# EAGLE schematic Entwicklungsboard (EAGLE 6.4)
Projekt einer Entwicklungsplatine. Designed vom Denys Maiier. Fakultät der Naturwissenschaften und Technik der HAWK Göttingen.

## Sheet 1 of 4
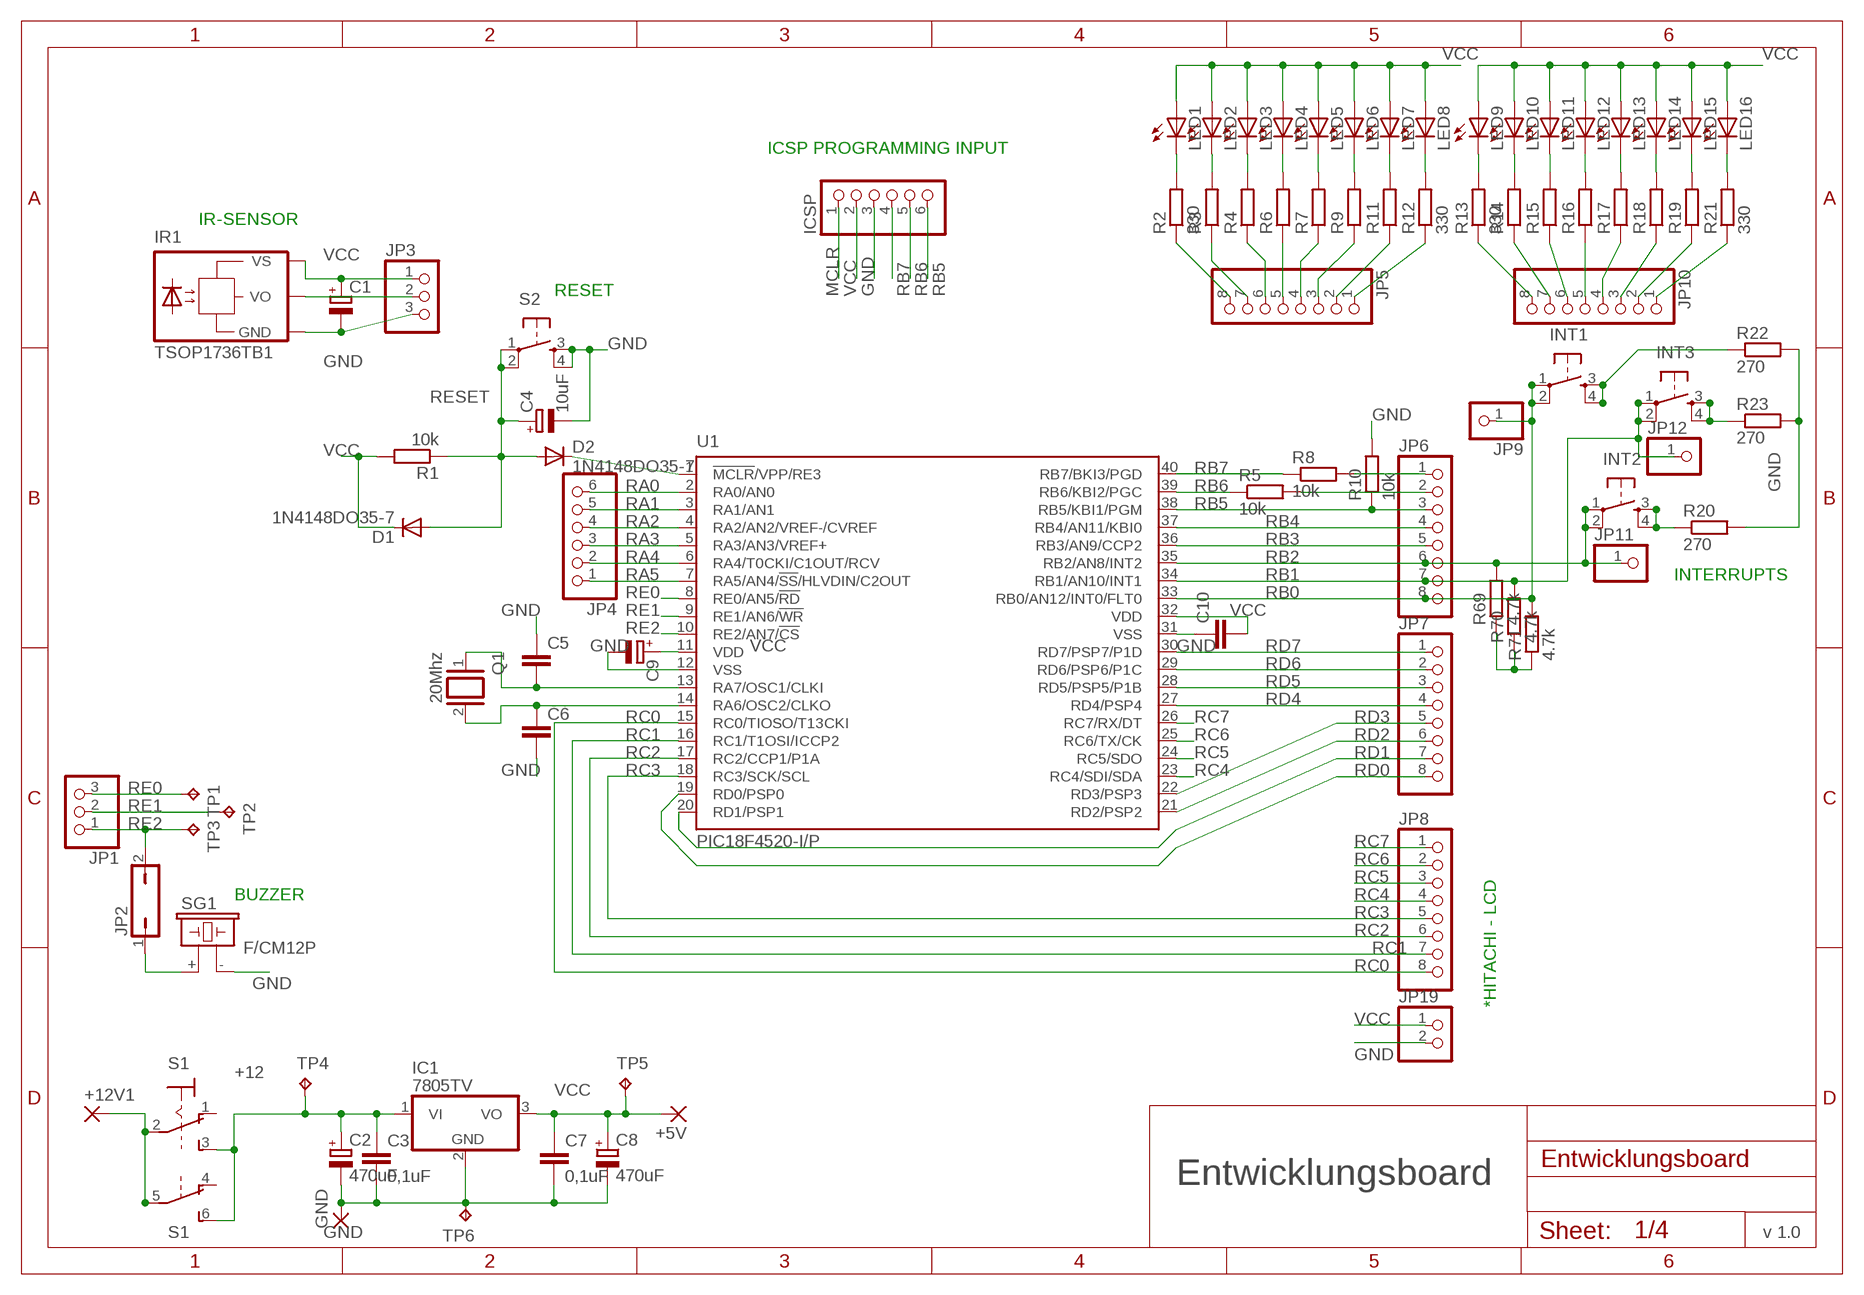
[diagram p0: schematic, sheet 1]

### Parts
+5V  2,15/1,0  [2,15/1,0]
+12V1  2,15/1,0  [2,15/1,0]
C1  CPOL-EUE2.5-5  [E2,5-5]
C2  470uF  CPOL-EUE7.5-16  [E7,5-16]
C3  0,1uF  C-EU075-042X103  [C075-042X103]
C4  10uF  CPOL-EUE2.5-6  [E2,5-6]
C5  C-EUC0805  [C0805]
C6  C-EUC0805  [C0805]
C7  0,1uF  C-EU075-042X103  [C075-042X103]
C8  470uF  CPOL-EUE7.5-16  [E7,5-16]
C9  CPOL-EUE3.5-8  [E3,5-8]
C10  C-EU050-025X075  [C050-025X075]
D1  1N4148DO35-7  [DO35-7]
D2  1N4148DO35-7  [DO35-7]
GND  2,15/1,0  [2,15/1,0]
IC1  7805TV  [TO220V]
ICSP  PINHD-1X6  [1X06]
INT1  10-XXB3FRAFI  [RAFI]
INT2  10-XXB3FRAFI  [RAFI]
INT3  10-XXB3FRAFI  [RAFI]
IR1  TSOP1736TB1  [TSOP17_TB1]
JP1  PINHD-1X3/90  [1X03/90]
JP2  JP1Q  [JP1]
JP3  PINHD-1X3  [1X03]
JP4  PINHD-1X6  [1X06]
JP5  PINHD-1X8  [1X08]
JP6  PINHD-1X8  [1X08]
JP7  PINHD-1X8  [1X08]
JP8  PINHD-1X8  [1X08]
JP9  PINHD-1X1  [1X01]
JP10  PINHD-1X8  [1X08]
JP11  PINHD-1X1  [1X01]
JP12  PINHD-1X1  [1X01]
JP19  PINHD-1X2  [1X02]
LED1  LED5MM  [LED5MM]
LED2  LED5MM  [LED5MM]
LED3  LED5MM  [LED5MM]
LED4  LED5MM  [LED5MM]
LED5  LED5MM  [LED5MM]
LED6  LED5MM  [LED5MM]
LED7  LED5MM  [LED5MM]
LED8  LED5MM  [LED5MM]
LED9  LED5MM  [LED5MM]
LED10  LED5MM  [LED5MM]
LED11  LED5MM  [LED5MM]
LED12  LED5MM  [LED5MM]
LED13  LED5MM  [LED5MM]
LED14  LED5MM  [LED5MM]
LED15  LED5MM  [LED5MM]
LED16  LED5MM  [LED5MM]
Q1  20Mhz  XTAL/S  [QS]
R1  10k  R-EU_M0805  [M0805]
R2  330  R-EU_M0805  [M0805]
R3  R-EU_M0805  [M0805]
R4  R-EU_M0805  [M0805]
R5  10k  R-EU_M0805  [M0805]
R6  R-EU_M0805  [M0805]
R7  R-EU_M0805  [M0805]
R8  10k  R-EU_M0805  [M0805]
R9  R-EU_M0805  [M0805]
R10  10k  R-EU_M0805  [M0805]
R11  R-EU_M0805  [M0805]
R12  330  R-EU_M0805  [M0805]
R13  330  R-EU_M0805  [M0805]
R14  R-EU_M0805  [M0805]
R15  R-EU_M0805  [M0805]
R16  R-EU_M0805  [M0805]
R17  R-EU_M0805  [M0805]
R18  R-EU_M0805  [M0805]
R19  R-EU_M0805  [M0805]
R20  270  R-EU_M0805  [M0805]
R21  330  R-EU_M0805  [M0805]
R22  270  R-EU_M0805  [M0805]
R23  270  R-EU_M0805  [M0805]
R69  4.7k  R-EU_M0805  [M0805]
R70  4.7k  R-EU_M0805  [M0805]
R71  4.7k  R-EU_M0805  [M0805]
S1  320-938  [320-938]
S2  10-XXB3FRAFI  [RAFI]
SG1  F/CM12P  [F/CM12P]
TP1  TPB2,54  [B2,54]
TP2  TPB2,54  [B2,54]
TP3  TPB2,54  [B2,54]
TP4  TPB2,54  [B2,54]
TP5  TPB2,54  [B2,54]
TP6  TPB2,54  [B2,54]
U1  PIC18F4520-I/P  [DIL40]

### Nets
+12: C2.+ C3.1 IC1.1(VI) S1.3(1:S) S1.6(B:S) TP4.TP
GND [GND]: C1.- C2.- C3.2 C4.- C5.1 C6.2 C7.2 C8.- C9.- C10.1 GND.1(P) IC1.2(GND) ICSP.3 IR1.GND JP3.3 JP19.2 R10.2 R20.2 R22.2 R23.2 S2.3(S) S2.4(S1) SG1.- TP6.TP U1.12(VSS) U1.31(VSS)
MCLR: D2.C ICSP.1 U1.1(!MCLR!/VPP/RE3)
N$1: C5.2 Q1.1 U1.13(RA7/OSC1/CLKI)
N$2: JP5.8 R2.1
N$3: C6.1 Q1.2 U1.14(RA6/OSC2/CLKO)
N$4: JP5.7 R3.1
N$5: JP10.8 R13.1
N$6: JP10.7 R14.1
N$7: JP10.6 R15.1
N$8: JP10.5 R16.1
N$9: JP10.4 R17.1
N$10: JP10.3 R18.1
N$11: JP10.2 R19.1
N$12: JP10.1 R21.1
N$13: LED9.K(C) R13.2
N$14: LED11.K(C) R15.2
N$15: LED12.K(C) R16.2
N$16: LED13.K(C) R17.2
N$17: LED16.K(C) R21.2
N$18: LED14.K(C) R18.2
N$19: LED10.K(C) R14.2
N$20: LED15.K(C) R19.2
N$21: JP5.6 R4.1
N$22: JP5.5 R6.1
N$23: JP5.4 R7.1
N$24: JP5.3 R9.1
N$25: JP5.2 R11.1
N$26: JP5.1 R12.1
N$27: LED1.K(C) R2.2
N$28: LED3.K(C) R4.2
N$29: LED4.K(C) R6.2
N$30: LED5.K(C) R7.2
N$31: LED8.K(C) R12.2
N$32: LED2.K(C) R3.2
N$33: LED6.K(C) R9.2
N$34: LED7.K(C) R11.2
N$48: INT1.3(S) INT1.4(S1) R22.1
N$57: JP6.1 R8.2
N$66: JP6.2 R5.2
N$118: INT2.3(S) INT2.4(S1) R20.1
N$122: JP2.1 SG1.+
N$137: IR1.VO JP3.2
N$160: INT3.3(S) INT3.4(S1) R23.1
N$163: +12V1.1(P) S1.2(1:P) S1.5(B:P)
RA0: JP4.6 U1.2(RA0/AN0)
RA1: JP4.5 U1.3(RA1/AN1)
RA2: JP4.4 U1.4(RA2/AN2/VREF-/CVREF)
RA3: JP4.3 U1.5(RA3/AN3/VREF+)
RA4: JP4.2 U1.6(RA4/T0CKI/C1OUT/RCV)
RA5: JP4.1 U1.7(RA5/AN4/!SS!/HLVDIN/C2OUT)
RB0: INT1.1(P) INT1.2(P1) JP6.8 JP9.1 R71.2 U1.33(RB0/AN12/INT0/FLT0)
RB1: INT3.1(P) INT3.2(P1) JP6.7 JP12.1 R70.2 U1.34(RB1/AN10/INT1)
RB2: INT2.1(P) INT2.2(P1) JP6.6 JP11.1 R69.2 U1.35(RB2/AN8/INT2)
RB3: JP6.5 U1.36(RB3/AN9/CCP2)
RB4: JP6.4 U1.37(RB4/AN11/KBI0)
RB5: ICSP.6 JP6.3 R10.1 U1.38(RB5/KBI1/PGM)
RB6: ICSP.5 R5.1 U1.39(RB6/KBI2/PGC)
RB7: ICSP.4 R8.1 U1.40(RB7/BKI3/PGD)
RC0: JP8.8 U1.15(RC0/TIOSO/T13CKI)
RC1: JP8.7 U1.16(RC1/T1OSI/ICCP2)
RC2: JP8.6 U1.17(RC2/CCP1/P1A)
RC3: JP8.5 U1.18(RC3/SCK/SCL)
RC4: JP8.4 U1.23(RC4/SDI/SDA)
RC5: JP8.3 U1.24(RC5/SDO)
RC6: JP8.2 U1.25(RC6/TX/CK)
RC7: JP8.1 U1.26(RC7/RX/DT)
RD0: JP7.8 U1.19(RD0/PSP0)
RD1: JP7.7 U1.20(RD1/PSP1)
RD2: JP7.6 U1.21(RD2/PSP2)
RD3: JP7.5 U1.22(RD3/PSP3)
RD4: JP7.4 U1.27(RD4/PSP4)
RD5: JP7.3 U1.28(RD5/PSP5/P1B)
RD6: JP7.2 U1.29(RD6/PSP6/P1C)
RD7: JP7.1 U1.30(RD7/PSP7/P1D)
RE0: JP1.3 TP1.TP U1.8(RE0/AN5/!RD)
RE1: JP1.2 TP2.TP U1.9(RE1/AN6/!WR)
RE2: JP1.1 JP2.2 TP3.TP U1.10(RE2/AN7/!CS)
RESET: C4.+ D1.A D2.A R1.1 S2.1(P) S2.2(P1)
VCC [VCC]: +5V.1(P) C1.+ C7.1 C8.+ C9.+ C10.2 D1.C IC1.3(VO) ICSP.2 IR1.VS JP3.1 JP19.1 LED1.A LED2.A LED3.A LED4.A LED5.A LED6.A LED7.A LED8.A LED9.A LED10.A LED11.A LED12.A LED13.A LED14.A LED15.A LED16.A R1.2 R69.1 R70.1 R71.1 TP5.TP U1.11(VDD) U1.32(VDD)
Unconnected: S1.1(1:O) S1.4(B:O)

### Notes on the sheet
- ICSP PROGRAMMING INPUT
- IR-SENSOR
- RESET
- INTERRUPTS
- BUZZER
- *HITACHI - LCD
- Entwicklungsboard
- v 1.0

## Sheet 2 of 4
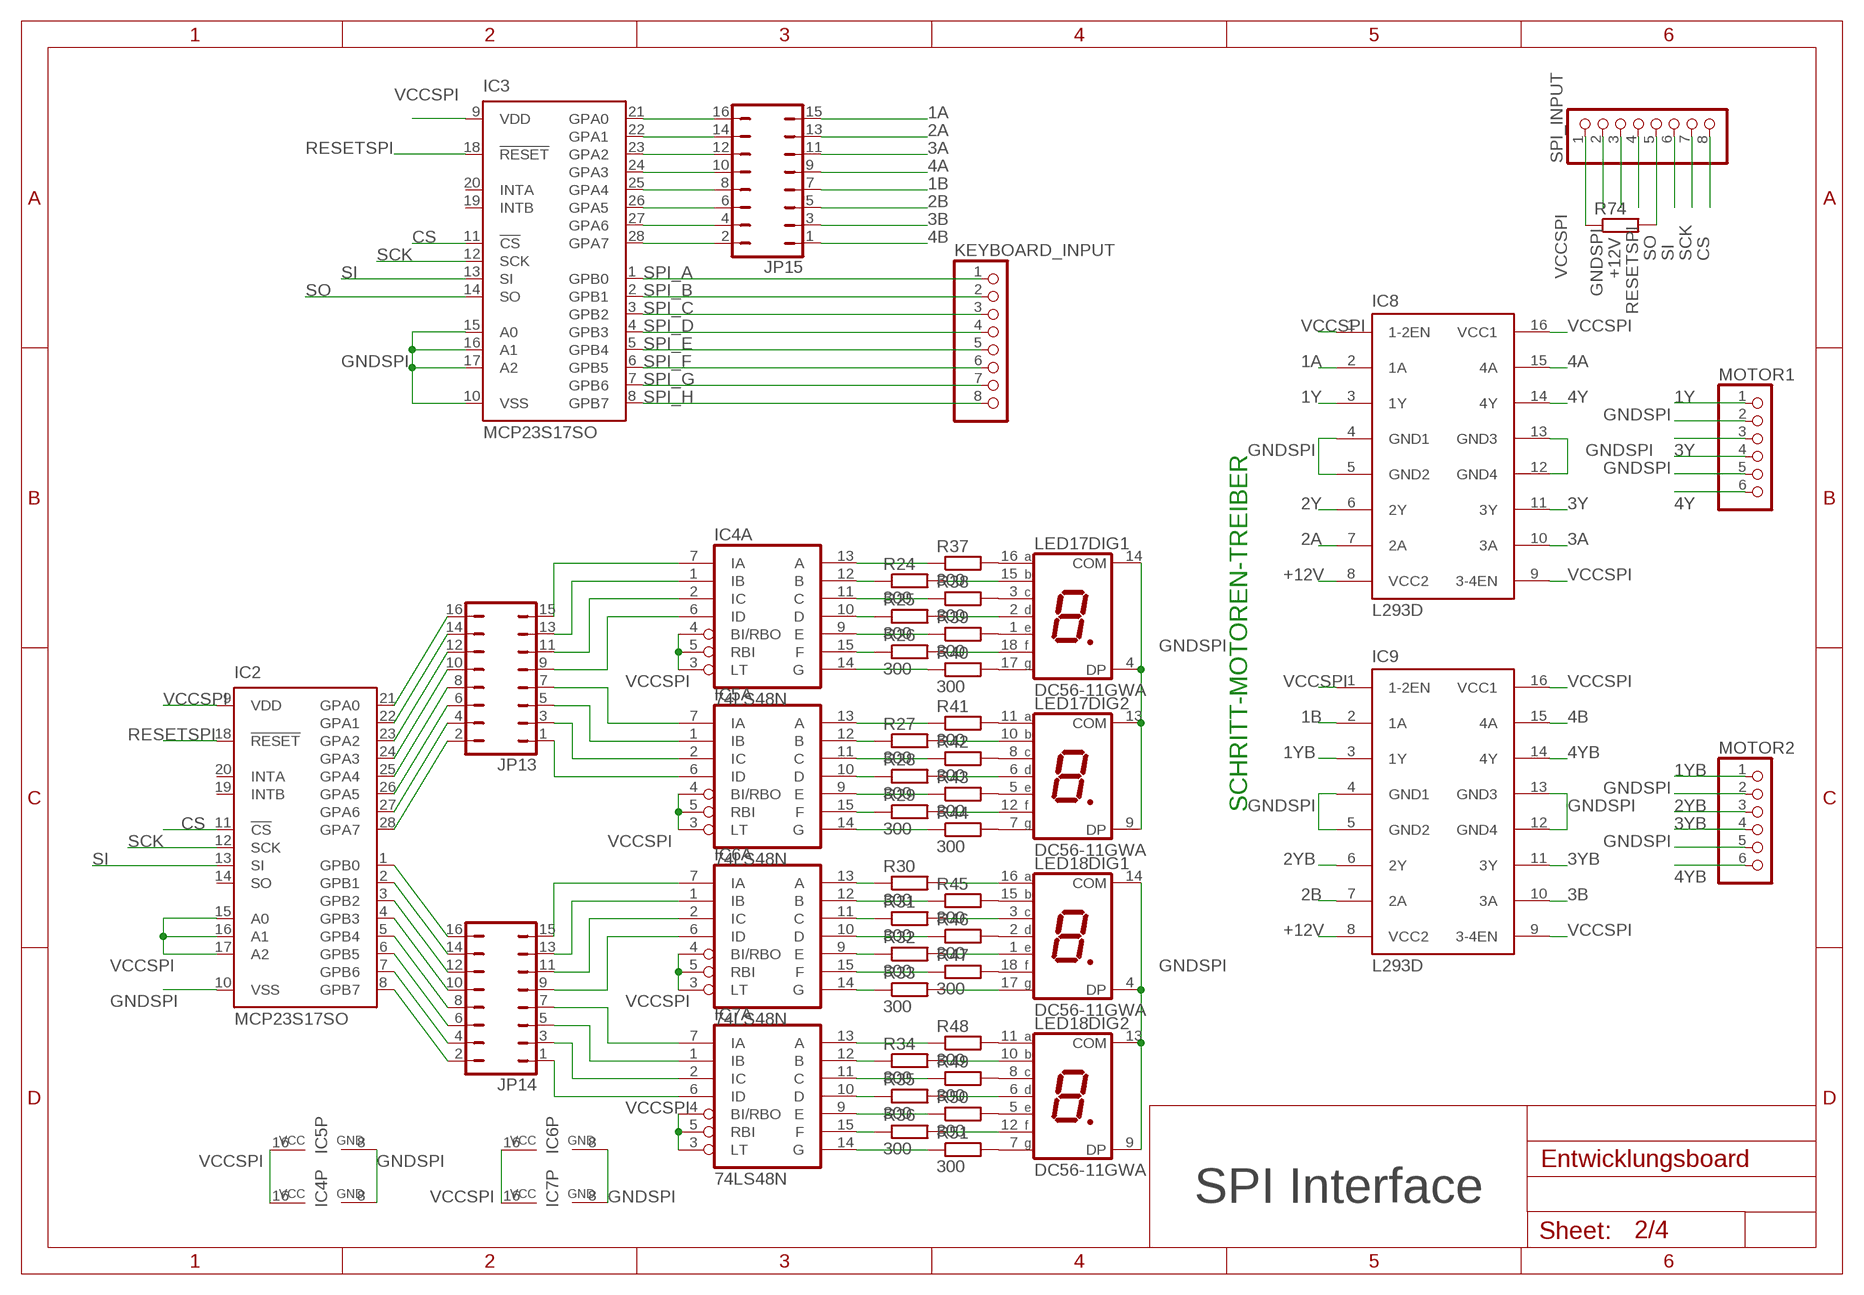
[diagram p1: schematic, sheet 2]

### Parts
IC2  MCP23S17SO  [SO28W]
IC3  MCP23S17SO  [SO28W]
IC4  74LS48N  [DIL16]
IC5  74LS48N  [DIL16]
IC6  74LS48N  [DIL16]
IC7  74LS48N  [DIL16]
IC8  L293D  [DIL16]
IC9  L293D  [DIL16]
JP13  JP8Q  [JP8Q]
JP14  JP8Q  [JP8Q]
JP15  JP8Q  [JP8Q]
KEYBOARD_INPUT  PINHD-1X8  [1X08]
LED17  DC56-11GWA  [DA56]
LED18  DC56-11GWA  [DA56]
MOTOR1  PINHD-1X6  [1X06]
MOTOR2  PINHD-1X6  [1X06]
R24  300  R-EU_R0805  [R0805]
R25  300  R-EU_R0805  [R0805]
R26  300  R-EU_R0805  [R0805]
R27  300  R-EU_R0805  [R0805]
R28  300  R-EU_R0805  [R0805]
R29  300  R-EU_R0805  [R0805]
R30  300  R-EU_R0805  [R0805]
R31  300  R-EU_R0805  [R0805]
R32  300  R-EU_R0805  [R0805]
R33  300  R-EU_R0805  [R0805]
R34  300  R-EU_R0805  [R0805]
R35  300  R-EU_R0805  [R0805]
R36  300  R-EU_R0805  [R0805]
R37  300  R-EU_R0805  [R0805]
R38  300  R-EU_R0805  [R0805]
R39  300  R-EU_R0805  [R0805]
R40  300  R-EU_R0805  [R0805]
R41  300  R-EU_R0805  [R0805]
R42  300  R-EU_R0805  [R0805]
R43  300  R-EU_R0805  [R0805]
R44  300  R-EU_R0805  [R0805]
R45  300  R-EU_R0805  [R0805]
R46  300  R-EU_R0805  [R0805]
R47  300  R-EU_R0805  [R0805]
R48  300  R-EU_R0805  [R0805]
R49  300  R-EU_R0805  [R0805]
R50  300  R-EU_R0805  [R0805]
R51  300  R-EU_R0805  [R0805]
R74  R-EU_M0805  [M0805]
SPI_INPUT  PINHD-1X8  [1X08]

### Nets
1A: IC8.2(1A) JP15.15
1B: IC9.2(1A) JP15.7
1Y: IC8.3(1Y) MOTOR1.1
1YB: IC9.3(1Y) MOTOR2.1
2A: IC8.7(2A) JP15.13
2B: IC9.7(2A) JP15.5
2Y: IC8.6(2Y) MOTOR1.3
2YB: IC9.6(2Y) MOTOR2.3
3A: IC8.10(3A) JP15.11
3B: IC9.10(3A) JP15.3
3Y: IC8.11(3Y) MOTOR1.4
3YB: IC9.11(3Y) MOTOR2.4
4A: IC8.15(4A) JP15.9
4B: IC9.15(4A) JP15.1
4Y: IC8.14(4Y) MOTOR1.6
4YB: IC9.14(4Y) MOTOR2.6
+12V: IC8.8(VCC2) IC9.8(VCC2) SPI_INPUT.3
CS: IC2.11(!CS) IC3.11(!CS) SPI_INPUT.8
GNDSPI: IC2.10(VSS) IC3.10(VSS) IC3.15(A0) IC3.16(A1) IC3.17(A2) IC4.8(P:GND) IC5.8(P:GND) IC6.8(P:GND) IC7.8(P:GND) IC8.4(GND1) IC8.5(GND2) IC8.12(GND4) IC8.13(GND3) IC9.4(GND1) IC9.5(GND2) IC9.12(GND4) IC9.13(GND3) LED17.4(DIG1:DP) LED17.9(DIG2:DP) LED17.13(DIG2:COM) LED17.14(DIG1:COM) LED18.4(DIG1:DP) LED18.9(DIG2:DP) LED18.13(DIG2:COM) LED18.14(DIG1:COM) MOTOR1.2 MOTOR1.5 MOTOR2.2 MOTOR2.5 SPI_INPUT.2
N$65: IC4.7(A:IA) JP13.15
N$67: IC4.1(A:IB) JP13.13
N$68: IC4.2(A:IC) JP13.11
N$69: IC4.6(A:ID) JP13.9
N$70: IC5.7(A:IA) JP13.7
N$71: IC5.1(A:IB) JP13.5
N$72: IC5.2(A:IC) JP13.3
N$73: IC5.6(A:ID) JP13.1
N$74: IC2.21(GPA0) JP13.16
N$75: IC2.22(GPA1) JP13.14
N$76: LED17.2(DIG1:D) R25.2
N$77: IC4.12(A:B) R24.1
N$78: IC4.13(A:A) R37.1
N$79: IC4.10(A:D) R25.1
N$80: IC4.11(A:C) R38.1
N$81: IC4.9(A:E) R39.1
N$82: IC4.15(A:F) R26.1
N$83: IC4.14(A:G) R40.1
N$84: IC5.13(A:A) R41.1
N$85: IC5.12(A:B) R27.1
N$86: IC5.11(A:C) R42.1
N$87: IC5.10(A:D) R28.1
N$88: IC5.9(A:E) R43.1
N$89: IC5.15(A:F) R29.1
N$90: IC5.14(A:G) R44.1
N$91: LED17.16(DIG1:A) R37.2
N$92: LED17.15(DIG1:B) R24.2
N$93: LED17.3(DIG1:C) R38.2
N$94: LED17.1(DIG1:E) R39.2
N$95: LED17.18(DIG1:F) R26.2
N$96: LED17.17(DIG1:G) R40.2
N$97: LED17.11(DIG2:A) R41.2
N$98: LED17.10(DIG2:B) R27.2
N$99: LED17.8(DIG2:C) R42.2
N$100: LED17.6(DIG2:D) R28.2
N$101: LED17.5(DIG2:E) R43.2
N$102: LED17.12(DIG2:F) R29.2
N$103: LED17.7(DIG2:G) R44.2
N$104: IC2.23(GPA2) JP13.12
N$105: IC2.24(GPA3) JP13.10
N$106: IC2.25(GPA4) JP13.8
N$107: IC2.26(GPA5) JP13.6
N$108: IC2.27(GPA6) JP13.4
N$109: IC2.28(GPA7) JP13.2
N$110: IC6.7(A:IA) JP14.15
N$111: IC6.1(A:IB) JP14.13
N$112: IC6.2(A:IC) JP14.11
N$113: IC6.6(A:ID) JP14.9
N$114: IC7.7(A:IA) JP14.7
N$115: IC7.1(A:IB) JP14.5
N$116: IC7.2(A:IC) JP14.3
N$117: IC7.6(A:ID) JP14.1
N$150: IC3.21(GPA0) JP15.16
N$151: IC3.22(GPA1) JP15.14
N$152: IC3.23(GPA2) JP15.12
N$153: IC3.24(GPA3) JP15.10
N$154: IC3.25(GPA4) JP15.8
N$155: IC3.26(GPA5) JP15.6
N$156: IC3.27(GPA6) JP15.4
N$157: IC3.28(GPA7) JP15.2
N$166: LED18.2(DIG1:D) R46.2
N$167: IC6.10(A:D) R46.1
N$168: IC6.13(A:A) R30.1
N$169: IC6.12(A:B) R45.1
N$170: IC6.11(A:C) R31.1
N$171: IC6.14(A:G) R33.1
N$172: IC6.15(A:F) R47.1
N$173: IC6.9(A:E) R32.1
N$174: IC7.13(A:A) R48.1
N$175: IC7.12(A:B) R34.1
N$176: IC7.11(A:C) R49.1
N$177: IC7.10(A:D) R35.1
N$178: IC7.9(A:E) R50.1
N$179: IC7.15(A:F) R36.1
N$180: IC7.14(A:G) R51.1
N$181: LED18.16(DIG1:A) R30.2
N$182: LED18.15(DIG1:B) R45.2
N$183: LED18.3(DIG1:C) R31.2
N$184: LED18.1(DIG1:E) R32.2
N$185: LED18.18(DIG1:F) R47.2
N$186: LED18.17(DIG1:G) R33.2
N$187: LED18.11(DIG2:A) R48.2
N$188: LED18.10(DIG2:B) R34.2
N$189: LED18.8(DIG2:C) R49.2
N$190: LED18.6(DIG2:D) R35.2
N$191: LED18.5(DIG2:E) R50.2
N$192: LED18.12(DIG2:F) R36.2
N$193: LED18.7(DIG2:G) R51.2
N$194: IC2.1(GPB0) JP14.16
N$195: IC2.2(GPB1) JP14.14
N$196: IC2.3(GPB2) JP14.12
N$197: IC2.4(GPB3) JP14.10
N$198: IC2.5(GPB4) JP14.8
N$199: IC2.6(GPB5) JP14.6
N$200: IC2.7(GPB6) JP14.4
N$201: IC2.8(GPB7) JP14.2
RESETSPI: IC2.18(!RESET) IC3.18(!RESET) SPI_INPUT.4
SCK: IC2.12(SCK) IC3.12(SCK) SPI_INPUT.7
SI: IC2.13(SI) IC3.13(SI) SPI_INPUT.6
SO: IC3.14(SO) R74.2 SPI_INPUT.5
SPI_A: IC3.1(GPB0) KEYBOARD_INPUT.1
SPI_B: IC3.2(GPB1) KEYBOARD_INPUT.2
SPI_C: IC3.3(GPB2) KEYBOARD_INPUT.3
SPI_D: IC3.4(GPB3) KEYBOARD_INPUT.4
SPI_E: IC3.5(GPB4) KEYBOARD_INPUT.5
SPI_F: IC3.6(GPB5) KEYBOARD_INPUT.6
SPI_G: IC3.7(GPB6) KEYBOARD_INPUT.7
SPI_H: IC3.8(GPB7) KEYBOARD_INPUT.8
VCCSPI: IC2.9(VDD) IC2.15(A0) IC2.16(A1) IC2.17(A2) IC3.9(VDD) IC4.3(A:LT) IC4.4(A:BI/RBO) IC4.5(A:RBI) IC4.16(P:VCC) IC5.3(A:LT) IC5.4(A:BI/RBO) IC5.5(A:RBI) IC5.16(P:VCC) IC6.3(A:LT) IC6.4(A:BI/RBO) IC6.5(A:RBI) IC6.16(P:VCC) IC7.3(A:LT) IC7.4(A:BI/RBO) IC7.5(A:RBI) IC7.16(P:VCC) IC8.1(1-2EN) IC8.9(3-4EN) IC8.16(VCC1) IC9.1(1-2EN) IC9.9(3-4EN) IC9.16(VCC1) R74.1 SPI_INPUT.1
Unconnected: IC2.14(SO) IC2.19(INTB) IC2.20(INTA) IC3.19(INTB) IC3.20(INTA)

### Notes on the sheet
- SCHRITT-MOTOREN-TREIBER
- SPI Interface

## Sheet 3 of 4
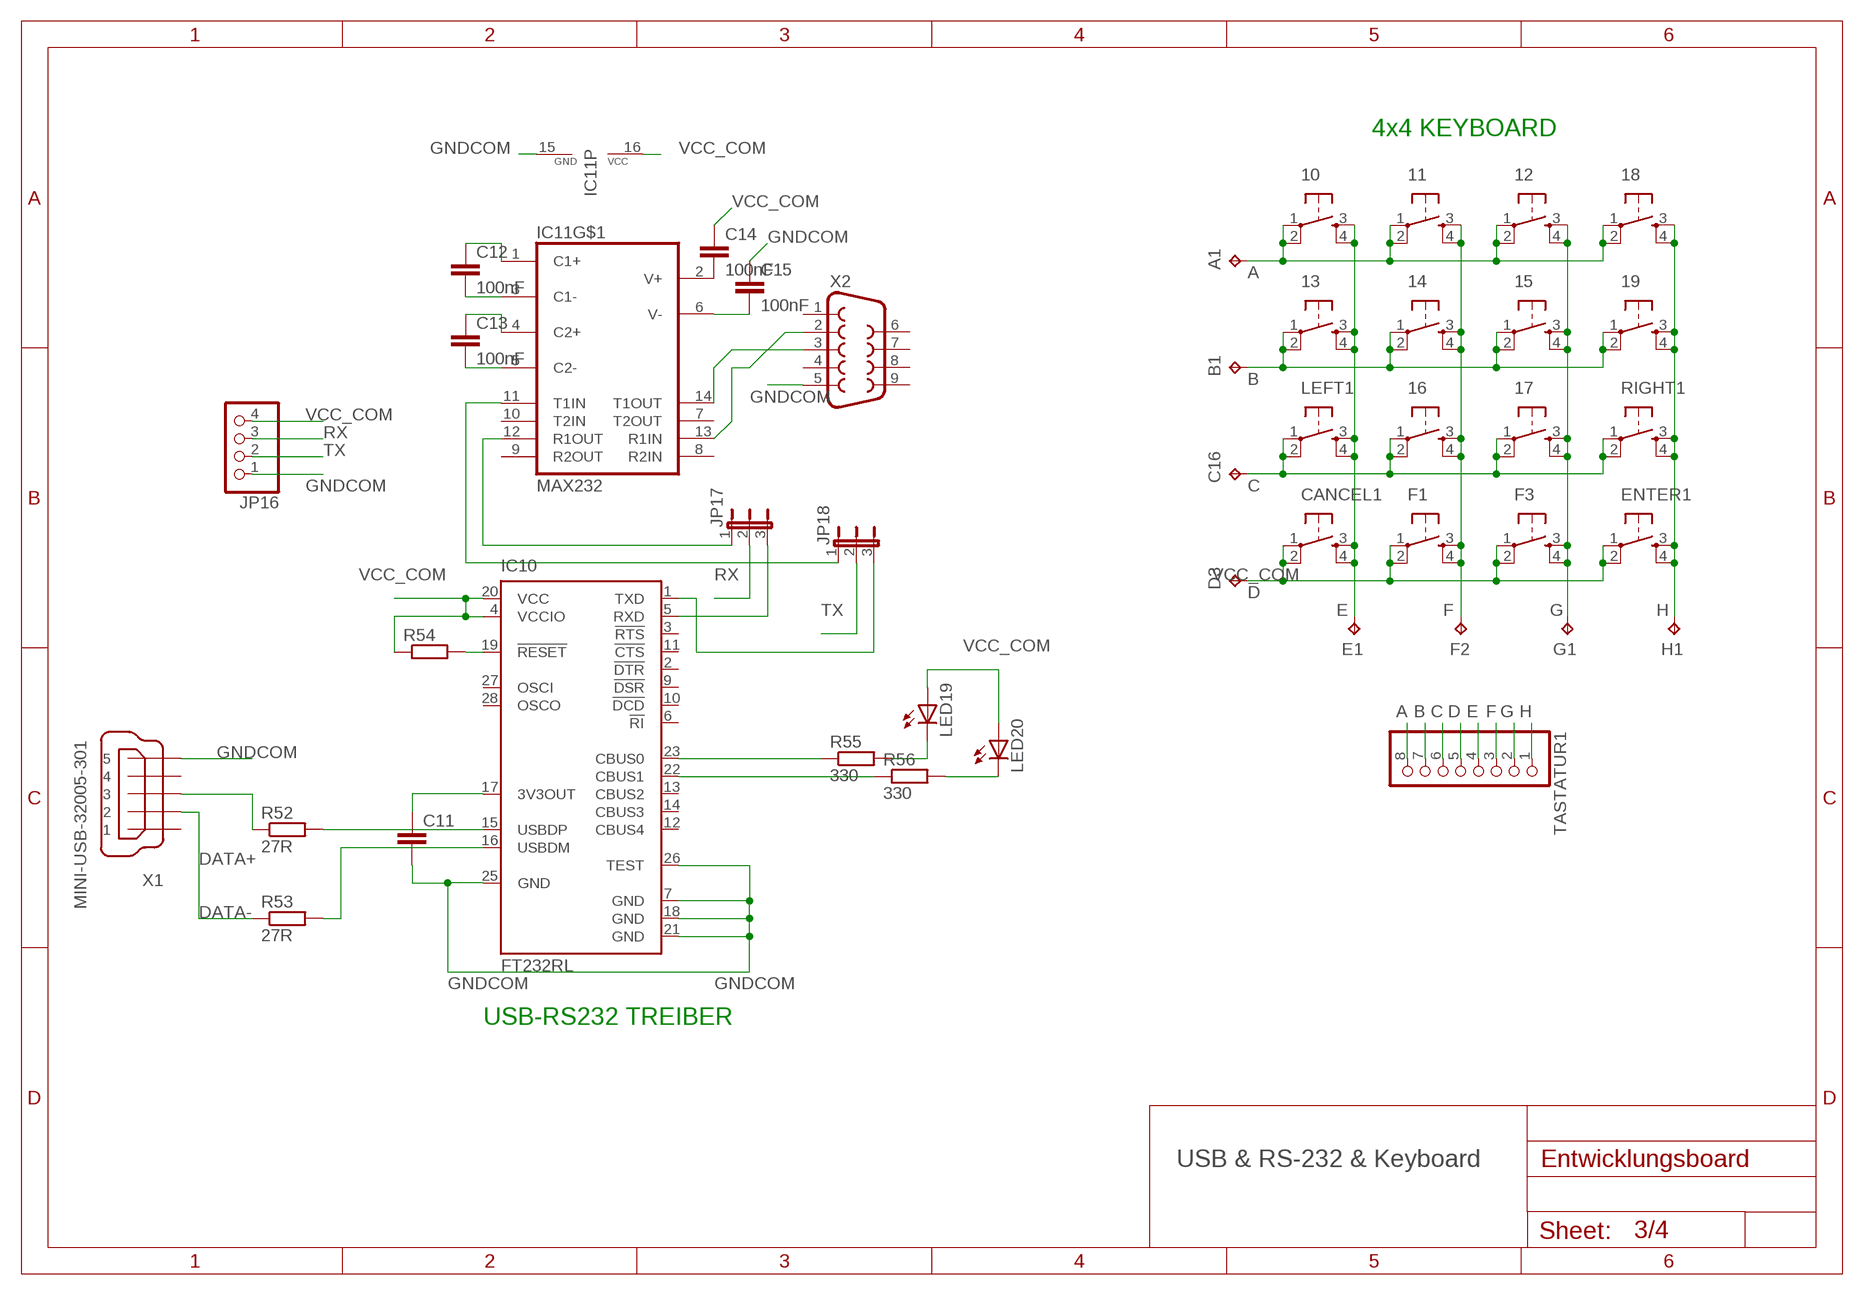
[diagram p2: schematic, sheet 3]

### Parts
10  10-XXB3FRAFI  [RAFI]
11  10-XXB3FRAFI  [RAFI]
12  10-XXB3FRAFI  [RAFI]
13  10-XXB3FRAFI  [RAFI]
14  10-XXB3FRAFI  [RAFI]
15  10-XXB3FRAFI  [RAFI]
16  10-XXB3FRAFI  [RAFI]
17  10-XXB3FRAFI  [RAFI]
18  10-XXB3FRAFI  [RAFI]
19  10-XXB3FRAFI  [RAFI]
A1  TPB2,54  [B2,54]
B1  TPB2,54  [B2,54]
C11  C-EUC0805  [C0805]
C12  100nF  C-EU075-032X103  [C075-032X103]
C13  100nF  C-EU075-032X103  [C075-032X103]
C14  100nF  C-EU075-032X103  [C075-032X103]
C15  100nF  C-EU075-032X103  [C075-032X103]
C16  TPB2,54  [B2,54]
CANCEL1  10-XXB3FRAFI  [RAFI]
D3  TPB2,54  [B2,54]
E1  TPB2,54  [B2,54]
ENTER1  10-XXB3FRAFI  [RAFI]
F1  10-XXB3FRAFI  [RAFI]
F2  TPB2,54  [B2,54]
F3  10-XXB3FRAFI  [RAFI]
G1  TPB2,54  [B2,54]
H1  TPB2,54  [B2,54]
IC10  FT232RL  [SSOP28]
IC11  MAX232  [DIL16]
JP16  PINHD-1X4  [1X04]
JP17  JP2E  [JP2]
JP18  JP2E  [JP2]
LED19  LED5MM  [LED5MM]
LED20  LED5MM  [LED5MM]
LEFT1  10-XXB3FRAFI  [RAFI]
R52  27R  R-EU_M0805  [M0805]
R53  27R  R-EU_M0805  [M0805]
R54  R-EU_M0805  [M0805]
R55  330  R-EU_M0805  [M0805]
R56  330  R-EU_M0805  [M0805]
RIGHT1  10-XXB3FRAFI  [RAFI]
TASTATUR1  PINHD-1X8  [1X08]
X1  MINI-USB-32005-301  [32005-301]
X2  F09H  [F09H]

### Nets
A: 10.1(P) 10.2(P1) 11.1(P) 11.2(P1) 12.1(P) 12.2(P1) 18.1(P) 18.2(P1) A1.TP TASTATUR1.8
B: 13.1(P) 13.2(P1) 14.1(P) 14.2(P1) 15.1(P) 15.2(P1) 19.1(P) 19.2(P1) B1.TP TASTATUR1.7
C: 16.1(P) 16.2(P1) 17.1(P) 17.2(P1) C16.TP LEFT1.1(P) LEFT1.2(P1) RIGHT1.1(P) RIGHT1.2(P1) TASTATUR1.6
D: CANCEL1.1(P) CANCEL1.2(P1) D3.TP ENTER1.1(P) ENTER1.2(P1) F1.1(P) F1.2(P1) F3.1(P) F3.2(P1) TASTATUR1.5
DATA+: R52.1 X1.3
DATA-: R53.1 X1.2
E: 10.3(S) 10.4(S1) 13.3(S) 13.4(S1) CANCEL1.3(S) CANCEL1.4(S1) E1.TP LEFT1.3(S) LEFT1.4(S1) TASTATUR1.4
F: 11.3(S) 11.4(S1) 14.3(S) 14.4(S1) 16.3(S) 16.4(S1) F1.3(S) F1.4(S1) F2.TP TASTATUR1.3
G: 12.3(S) 12.4(S1) 15.3(S) 15.4(S1) 17.3(S) 17.4(S1) F3.3(S) F3.4(S1) G1.TP TASTATUR1.2
GNDCOM: C11.2 C15.1 IC10.7(GND) IC10.18(GND) IC10.21(GND) IC10.25(GND) IC10.26(TEST) IC11.15(P:GND) JP16.1 X1.5 X2.5
H: 18.3(S) 18.4(S1) 19.3(S) 19.4(S1) ENTER1.3(S) ENTER1.4(S1) H1.TP RIGHT1.3(S) RIGHT1.4(S1) TASTATUR1.1
N$35: IC11.14(T1OUT) X2.3
N$36: IC11.13(R1IN) X2.2
N$37: C14.2 IC11.2(V+)
N$38: C15.2 IC11.6(V-)
N$39: C12.2 IC11.3(C1-)
N$40: C12.1 IC11.1(C1+)
N$41: C13.1 IC11.4(C2+)
N$42: C13.2 IC11.5(C2-)
N$43: IC10.22(CBUS1) R56.1
N$44: IC10.23(CBUS0) R55.1
N$45: LED19.K(C) R55.2
N$46: LED20.K(C) R56.2
N$47: C11.1 IC10.17(3V3OUT)
N$49: IC10.15(USBDP) R52.2
N$52: IC10.1(TXD) JP18.3
N$55: IC10.16(USBDM) R53.2
N$56: IC11.11(T1IN) JP18.1
N$58: IC10.5(RXD) JP17.3
N$59: IC11.12(R1OUT) JP17.1
N$64: IC10.19(!RESET) R54.2
RX: JP16.3 JP17.2
TX: JP16.2 JP18.2
VCC_COM: C14.1 IC10.4(VCCIO) IC10.20(VCC) IC11.16(P:VCC) JP16.4 LED19.A LED20.A R54.1
Unconnected: IC10.2(!DTR) IC10.3(!RTS) IC10.6(!RI) IC10.9(!DSR) IC10.10(!DCD) IC10.11(!CTS) IC10.12(CBUS4) IC10.13(CBUS2) IC10.14(CBUS3) IC10.27(OSCI) IC10.28(OSCO) IC11.7(T2OUT) IC11.8(R2IN) IC11.9(R2OUT) IC11.10(T2IN) X1.1 X1.4 X2.1 X2.4 X2.6 X2.7 X2.8 X2.9

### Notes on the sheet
- 4x4 KEYBOARD
- USB-RS232 TREIBER
- USB & RS-232 & Keyboard

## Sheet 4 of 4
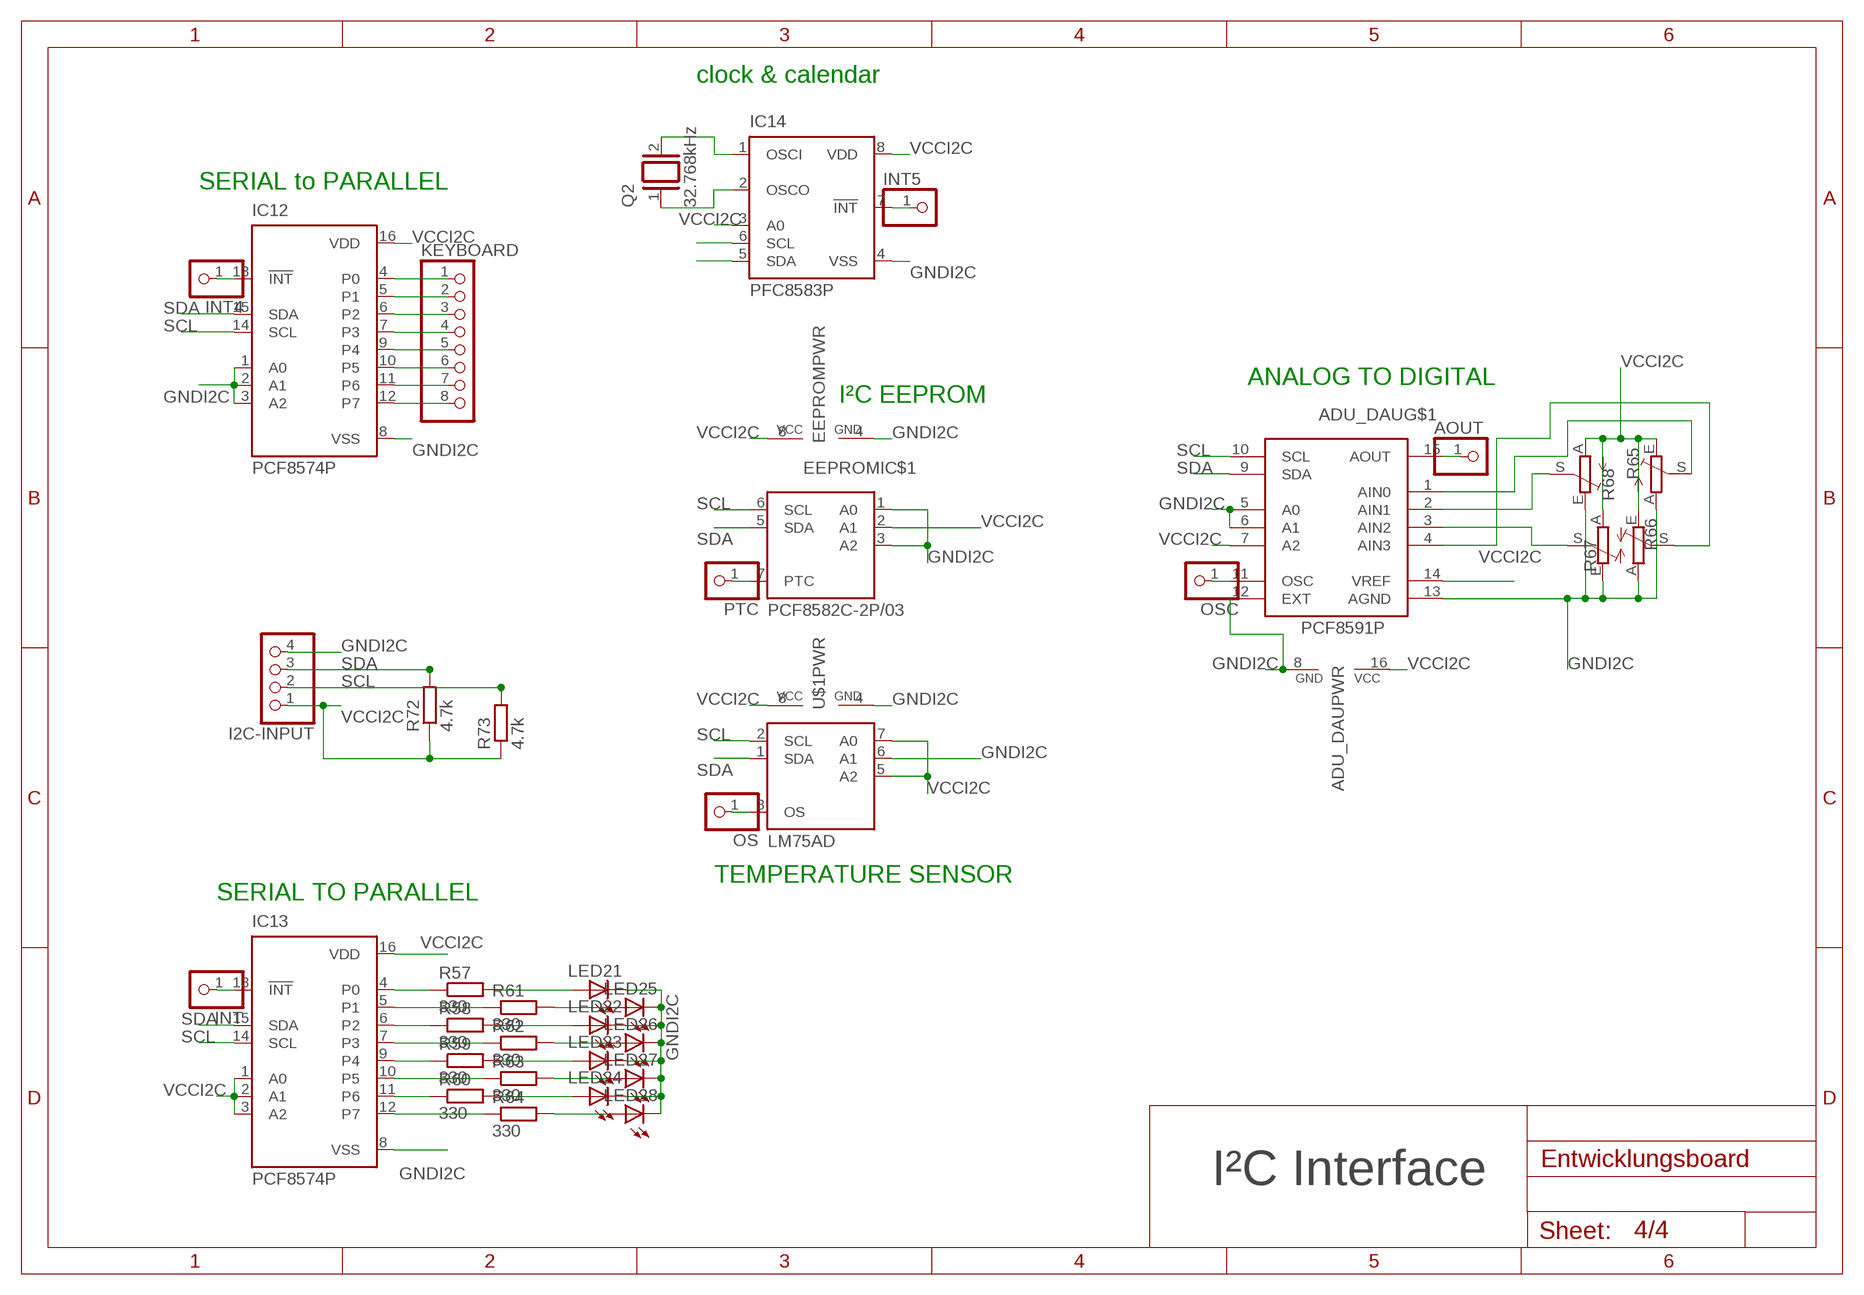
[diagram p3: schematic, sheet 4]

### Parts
ADU_DAU  PCF8591P  [DIL16]
AOUT  PINHD-1X1  [1X01]
EEPROM  PCF8582C-2P/03  [DIL08]
I2C-INPUT  PINHD-1X4  [1X04]
IC12  PCF8574P  [DIL16]
IC13  PCF8574P  [DIL16]
IC14  PFC8583P  [DIL08]
INT  PINHD-1X1  [1X01]
INT4  PINHD-1X1  [1X01]
INT5  PINHD-1X1  [1X01]
KEYBOARD  PINHD-1X8  [1X08]
LED21  LED5MM  [LED5MM]
LED22  LED5MM  [LED5MM]
LED23  LED5MM  [LED5MM]
LED24  LED5MM  [LED5MM]
LED25  LED5MM  [LED5MM]
LED26  LED5MM  [LED5MM]
LED27  LED5MM  [LED5MM]
LED28  LED5MM  [LED5MM]
OS  PINHD-1X1  [1X01]
OSC  PINHD-1X1  [1X01]
PTC  PINHD-1X1  [1X01]
Q2  32.768kHz  XTAL/S  [QS]
R57  330  R-EU_M0805  [M0805]
R58  330  R-EU_M0805  [M0805]
R59  330  R-EU_M0805  [M0805]
R60  330  R-EU_M0805  [M0805]
R61  330  R-EU_M0805  [M0805]
R62  330  R-EU_M0805  [M0805]
R63  330  R-EU_M0805  [M0805]
R64  330  R-EU_M0805  [M0805]
R65  TRIM_EU-CIP20C-6MM  [CIP20C-6MM]
R66  TRIM_EU-CIP20C-6MM  [CIP20C-6MM]
R67  TRIM_EU-CIP20C-6MM  [CIP20C-6MM]
R68  TRIM_EU-CIP20C-6MM  [CIP20C-6MM]
R72  4.7k  R-EU_M0805  [M0805]
R73  4.7k  R-EU_M0805  [M0805]
U$1  LM75AD  [SO08]

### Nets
GNDI2C: ADU_DAU.5(A0) ADU_DAU.6(A1) ADU_DAU.8(PWR:GND) ADU_DAU.12(EXT) ADU_DAU.13(AGND) EEPROM.1(IC$1:A0) EEPROM.3(IC$1:A2) EEPROM.4(PWR:GND) I2C-INPUT.4 IC12.1(A0) IC12.2(A1) IC12.3(A2) IC12.8(VSS) IC13.8(VSS) IC14.4(VSS) LED21.K(C) LED22.K(C) LED23.K(C) LED24.K(C) LED25.K(C) LED26.K(C) LED27.K(C) LED28.K(C) R65.E R66.E R67.A R68.A U$1.4(PWR:GND) U$1.6(IC$1:A1)
N$50: IC12.4(P0) KEYBOARD.1
N$51: IC12.5(P1) KEYBOARD.2
N$53: IC12.6(P2) KEYBOARD.3
N$54: IC12.7(P3) KEYBOARD.4
N$60: IC12.9(P4) KEYBOARD.5
N$61: IC12.10(P5) KEYBOARD.6
N$62: IC12.11(P6) KEYBOARD.7
N$63: IC12.12(P7) KEYBOARD.8
N$162: IC13.4(P0) R57.1
N$164: IC13.5(P1) R61.1
N$213: IC13.6(P2) R58.1
N$214: IC13.7(P3) R62.1
N$215: IC13.9(P4) R59.1
N$216: IC13.10(P5) R63.1
N$217: IC13.11(P6) R60.1
N$218: IC13.12(P7) R64.1
N$219: LED21.A R57.2
N$220: LED25.A R61.2
N$221: LED22.A R58.2
N$222: LED26.A R62.2
N$223: LED23.A R59.2
N$224: LED27.A R63.2
N$225: LED24.A R60.2
N$226: LED28.A R64.2
N$227: ADU_DAU.11(OSC) OSC.1
N$228: IC14.1(OSCI) Q2.2
N$229: EEPROM.7(IC$1:PTC) PTC.1
N$230: OS.1 U$1.3(IC$1:OS)
N$231: ADU_DAU.15(AOUT) AOUT.1
N$232: IC14.2(OSCO) Q2.1
N$233: IC13.13(!INT) INT.1
N$234: IC12.13(!INT) INT4.1
N$235: IC14.7(!INT) INT5.1
N$236: ADU_DAU.2(AIN1) R65.S
N$237: ADU_DAU.3(AIN2) R66.S
N$238: ADU_DAU.1(AIN0) R68.S
N$239: ADU_DAU.4(AIN3) R67.S
SCL: ADU_DAU.10(SCL) EEPROM.6(IC$1:SCL) I2C-INPUT.2 IC12.14(SCL) IC13.14(SCL) IC14.6(SCL) R73.2 U$1.2(IC$1:SCL)
SDA: ADU_DAU.9(SDA) EEPROM.5(IC$1:SDA) I2C-INPUT.3 IC12.15(SDA) IC13.15(SDA) IC14.5(SDA) R72.2 U$1.1(IC$1:SDA)
VCCI2C: ADU_DAU.7(A2) ADU_DAU.14(VREF) ADU_DAU.16(PWR:VCC) EEPROM.2(IC$1:A1) EEPROM.8(PWR:VCC) I2C-INPUT.1 IC12.16(VDD) IC13.1(A0) IC13.2(A1) IC13.3(A2) IC13.16(VDD) IC14.3(A0) IC14.8(VDD) R65.A R66.A R67.E R68.E R72.1 R73.1 U$1.5(IC$1:A2) U$1.7(IC$1:A0) U$1.8(PWR:VCC)

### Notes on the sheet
- clock & calendar
- SERIAL to PARALLEL
- ANALOG TO DIGITAL
- I²C EEPROM
- TEMPERATURE SENSOR
- SERIAL TO PARALLEL
- I²C Interface

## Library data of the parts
10-19 CANCEL1 ENTER1 F1 F3 INT1-INT3 LEFT1 RIGHT1 S2 = switch-omron:10-XX: OMRON SWITCH
+5V +12V1 GND = wirepad:2,15/1,0: THROUGH-HOLE PAD
A1 B1 C16 D3 E1 F2 G1 H1 TP1-TP6 = testpad:TP: Test pad
ADU_DAU = i2c:PCF8591: 8-Bit A/D and D/A Converter
AOUT INT INT4 INT5 JP9 JP11 JP12 OS OSC PTC = pinhead:PINHD-1X1: PIN HEADER
C1 C2 C4 C8 C9 = rcl:CPOL-EU: POLARIZED CAPACITOR, European symbol
C3 C5-C7 C10-C15 = rcl:C-EU: CAPACITOR, European symbol
D1 D2 = diode:1N4148: DIODE
EEPROM = i2c:PCF8582C-2: 256 x 8-Bit CMOS EEPROM with I²C Bus Interface
I2C-INPUT JP16 = pinhead:PINHD-1X4: PIN HEADER
IC1 = linear:78*: Positive VOLTAGE REGULATOR Source: http://cache.national.com/ds/LM/LM78L05.pdf http://www.fairchildsemi.com/ds/LM/LM7805.pdf
IC2 IC3 = microchip:MCP23S17: http://ww1.microchip.com/downloads/en/DeviceDoc/21952a.pdf Source: http://ww1.microchip.com/downloads/en/DeviceDoc/21952a.pdf; MF: MICROCHIP; MPN: MCP23S17-E/SO; OC_FARNELL: unknown; OC_NEWARK: 31K2950
IC4-IC7 = 74xx-eu:74*48: BCD to seven segment DECODER/DRIVER
IC8 IC9 = st-microelectronics:L293D: PUSH-PULL 4 CHANNEL DRIVER; MPN: L293D; OC_FARNELL: 9589619; OC_NEWARK: 56P8249
IC10 = ftdichip:FT232R: Source: http://www.ftdichip.com/Documents/DataSheets/DS_FT232R_v104.pdf; MPN: FT232RL; OC_FARNELL: 1146032; OC_NEWARK: 91K9918
IC11 = maxim:MAX232: RS232 TRANSEIVER; MF: MAXIM; MPN: MAX232ACPE+; OC_FARNELL: 9723773; OC_NEWARK: 68K4544
IC12 IC13 = micro-philips:PCF8574: I2C-Bus Remote 8-bit I/O expander http://www.semiconductors.philips.com/acrobat_download/datasheets/PCF8574_4.pdf; MPN: PCF8574PN; OC_FARNELL: 204020; OC_NEWARK: 11N8515
IC14 = micro-philips:PFC8583: I2C-Bus CLOCK/CALENDAR; OC_FARNELL: unknown; OC_NEWARK: unknown
ICSP JP4 MOTOR1 MOTOR2 = pinhead:PINHD-1X6: PIN HEADER
IR1 = telefunken:TSOP17*TB1: TSOP17..TB1 IR Receiver Modules for Remote Control Systems Source: http://www.vishay.com/docs/82042/82042.pdf; OC_FARNELL: unknown; OC_NEWARK: unknown
JP1 JP3 = pinhead:PINHD-1X3: PIN HEADER
JP2 = jumper:JP1Q: JUMPER
JP5-JP8 JP10 KEYBOARD KEYBOARD_INPUT SPI_INPUT TASTATUR1 = pinhead:PINHD-1X8: PIN HEADER
JP13-JP15 = jumper:JP8Q: JUMPER
JP17 JP18 = jumper:JP2E: JUMPER
JP19 = pinhead:PINHD-1X2: PIN HEADER
LED1-LED16 LED19-LED28 = led:LED: LED
LED17 LED18 = display-kingbright-1:DC56-11: 14.22mm (0.56INCH) DUAL DIGIT NUMERIC DISPLAYS Source: www.kingbright.com .. DA56-11SRWA.pdf
Q1 Q2 = special:XTAL/S: CRYSTAL
R1 = resistor:R-EU_: RESISTOR, European symbol
R2-R64 R69-R74 = rcl:R-EU_: RESISTOR, European symbol
R65-R68 = pot:TRIM_EU-: POTENTIOMETER
S1 = switch:320-938: TOGGLE SWITCH distributor RS Components
SG1 = buzzer:F/CM12P: BUZZER; OC_FARNELL: unknown; OC_NEWARK: unknown
U1 = microchip-pic18:PIC18F4*20: Microcontrollers with nanoWatt Technology High-Performance, Enhanced Flash, 28/40/44-Pin,
U$1 = i2c:LM75AD: Digital Temperature Sensor and Thermal Watchdog
X1 = con-cypressindustries:MINI-USB-: MINI USB-B Conector Source: www.cypressindustries.com; OC_FARNELL: unknown; OC_NEWARK: unknown
X2 = con-subd:F09: SUB-D; OC_FARNELL: unknown; OC_NEWARK: unknown

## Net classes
0 default: width 0.3 mm
1 GND: width 0.8 mm
2 VCC: width 0.8 mm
